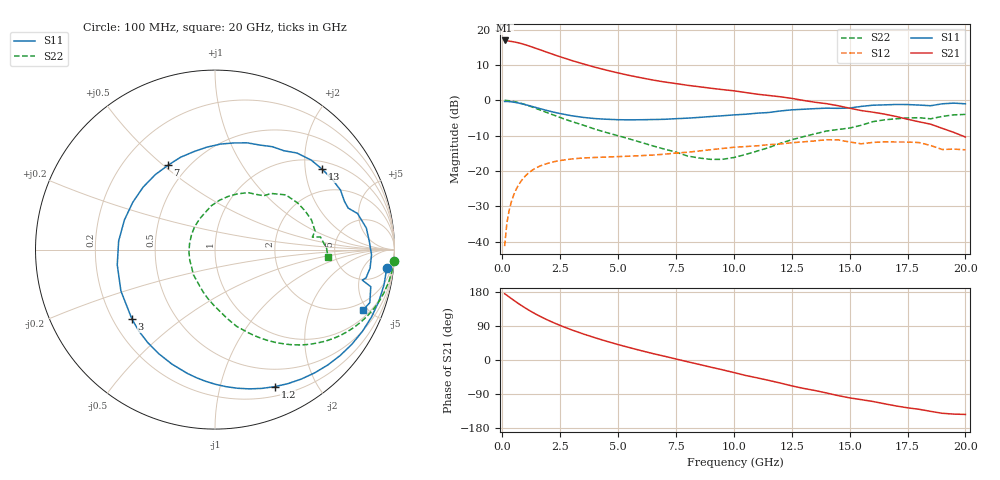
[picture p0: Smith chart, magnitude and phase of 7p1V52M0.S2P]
! Infineon Technologies  Discrete & RF Semiconductors
! bfp620
! VCE =  1.5 V,  IC =  2.0 mA
! Common Emitter S-Parameters:  Sep 2002
# GHz  S  MA  R  50
!  f  S11  S21  S12  S22
! GHz  MAG  ANG  MAG  ANG  MAG  ANG  MAG  ANG
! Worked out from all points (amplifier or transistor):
!   59 points, 100 MHz to 20 GHz, reference 50 ohm
!   highest |S21| = 16.9 dB at 100 MHz (marker M1)
!   |S21| within 3 dB of that: start of sweep to 1.787 GHz
!   unconditionally stable (mu >= 1): 5.822 GHz to 13.95 GHz; 14.03 GHz to 15.7 GHz; 17.5 GHz to end of sweep
!   at 1 GHz: K = 0.16, MSG = 18.6 dB, |S12| = -21.4 dB
!   at 5.5 GHz: K = 0.96, MSG = 11.4 dB, |S12| = -15.8 dB
!   at 20 GHz: K = 1.45, MAG = -2.2 dB, |S12| = -14.0 dB
!   S11 on the Smith chart (normalised r, x): 100 MHz: 6, -17; 1.2 GHz: 0.30, -1.49; 3 GHz: 0.28, -0.34; 7 GHz: 0.39, +0.52; 13 GHz: 1.22, +2.47; 20 GHz: 1.44, -4.72
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0.1  0.9626 -6.1  7.035 174.9  0.0086 86.7  0.9982 -3.5
0.3  0.9573 -17.5  6.884 166.2  0.028 80.3  0.9851 -10.4
0.5  0.9393 -29.0  6.717 157.3  0.0463 73.6  0.9606 -17.1
0.7  0.9136 -40.2  6.505 148.9  0.0631 66.8  0.9273 -23.3
1  0.8669 -56.3  6.103 137.0  0.085 57.2  0.8667 -31.9
1.2  0.8332 -66.4  5.809 129.7  0.0972 51.4  0.8228 -37.1
1.6  0.7665 -85.3  5.232 116.2  0.1161 41.3  0.7355 -46.0
2  0.7071 -102.5  4.705 104.4  0.1292 33.1  0.6566 -53.3
2.4  0.6592 -118.4  4.236 93.7  0.1385 26.3  0.5872 -59.7
3  0.6034 -140.1  3.659 79.4  0.1476 17.8  0.5005 -68.0
3.5  0.5726 -156.3  3.272 68.7  0.1526 12.0  0.4441 -74.3
4  0.5512 -171.1  2.942 58.8  0.1551 7.1  0.3906 -79.9
5  0.5311 161.9  2.44 40.7  0.1595 0.2  0.315 -90.4
6  0.5306 139.0  2.082 24.6  0.1646 -5.2  0.2536 -103.5
7  0.5379 119.1  1.818 10.0  0.1723 -9.3  0.2038 -119.0
8.5  0.5725 94.6  1.557 -11.6  0.1916 -16.7  0.1523 -157.4
10.5  0.6344 66.6  1.29 -40.7  0.2212 -30.9  0.1705 131.8
13  0.7465 36.8  0.996 -74.8  0.2581 -49.7  0.3053 76.1
13.5  0.7616 31.1  0.939 -80.5  0.2659 -54.3  0.3347 68.1
15  0.7773 17.3  0.773 -99.9  0.257 -74.0  0.4047 47.8
17  0.8724 -1.9  0.591 -121.2  0.2568 -86.1  0.5472 23.0
20  0.8923 -22.0  0.302 -143.6  0.1991 -107.7  0.631 -3.9
